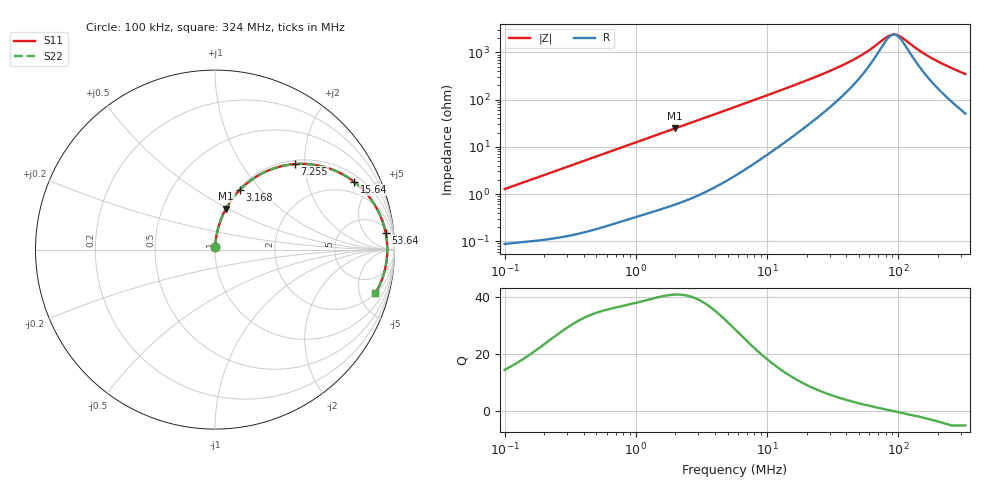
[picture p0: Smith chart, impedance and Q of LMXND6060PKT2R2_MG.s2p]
! LMXND6060PKT2R2_MG  S-PARAMETER MODEL  ( General Type )
! Model Generated by TAIYO YUDEN Corporation (https://www.yuden.co.jp/en/)
! Version 1.0
! TAIYO YUDEN Control No. 191025NI43SB-FBB
! Copyright(c) 2019 TAIYO YUDEN CO.,LTD. All Rights Reserved.
! Product Description (link to TY-COMPAS)
! https://ds.yuden.co.jp/TYCOMPAS/or/detail?pn=LMXND6060PKT2R2NMG&u=M
! Products Name : Inductors
! Characteristics :
!  Inductance : 2.2 uH , SRF(min) : 61 MHz , DC Resistance(max) : 0.066 Ohm
!  Rated Current : Saturation :3000 mA , Temp Rise : 2300 mA (40 degC)
!  Case Size : 6.0 x 6.0 / 0.236 x 0.236 [mm/inch] , Thickness : 1.4 / 0.055 [mm/inch]
!  (Conditions: Temperature = 25 degC , DC Bias Current/Voltage = 0A / 0V)
! External Node Assignments :
!  1  o---GGG---o  2
! GND o---------o GND
! Frequency Range : 0.1MHz  -  324.04089MHz  [ 402 STEP ]
# MHz S RI R 50
! Freq[MHz].  S11 Real  S11 Imag  S21 Real  S21 Imag  S12 Real  S12 Imag  S22 Real  S22 Imag
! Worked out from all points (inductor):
!   401 points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, 100 kHz to 324 MHz, reference 50 ohm
!   read as one part in series: L = 2.02 uH near 104.1 kHz
!   highest Q = 40.9 at 1.99 MHz (marker M1), where L = 1.95 uH
!   self-resonance near 92.57 MHz
!   S11 on the Smith chart (normalised r, x): 100 kHz: 1.00, +0.03; 3.168 MHz: 1.02, +0.78; 7.255 MHz: 1.07, +1.78; 15.64 MHz: 1.33, +3.91; 53.64 MHz: 8, +17; 324 MHz: 2.01, -6.89
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0.1  0.00104 0.0127  0.999 -0.0127  0.999 -0.0127  0.00104 0.0127
0.38728  0.00383 0.0482  0.9962 -0.0482  0.9962 -0.0482  0.00383 0.0482
0.80164  0.0124 0.098  0.9876 -0.098  0.9876 -0.098  0.0124 0.098
1.499861  0.0371 0.177  0.9629 -0.177  0.9629 -0.177  0.0371 0.177
1.990316  0.0613 0.228  0.9387 -0.228  0.9387 -0.228  0.0613 0.228
3.167973  0.1373 0.3315  0.8627 -0.3315  0.8627 -0.3315  0.1373 0.3315
4.2039  0.2164 0.3976  0.7836 -0.3976  0.7836 -0.3976  0.2164 0.3976
5.692459  0.3332 0.4543  0.6668 -0.4543  0.6668 -0.4543  0.3332 0.4543
7.254674  0.4451 0.4766  0.5549 -0.4766  0.5549 -0.4766  0.4451 0.4766
10.22865  0.609 0.4608  0.391 -0.4608  0.391 -0.4608  0.609 0.4608
15.63597  0.7748 0.3778  0.2252 -0.3778  0.2252 -0.3778  0.7748 0.3778
22.04577  0.8622 0.2897  0.1378 -0.2897  0.1378 -0.2897  0.8622 0.2897
36.53742  0.9292 0.1686  0.0708 -0.1686  0.0708 -0.1686  0.9292 0.1686
53.64032  0.9509 0.0925  0.0491 -0.0925  0.0491 -0.0925  0.9509 0.0925
85.37896  0.9598 0.0132  0.0402 -0.0132  0.0402 -0.0132  0.9598 0.0132
92.56714  0.96 9.66e-06  0.04 -9.66e-06  0.04 -9.66e-06  0.96 9.66e-06
100.3605  0.9598 -0.0132  0.0402 0.0132  0.0402 0.0132  0.9598 -0.0132
108.81  0.9593 -0.0264  0.0407 0.0264  0.0407 0.0264  0.9593 -0.0264
144.3909  0.9542 -0.0744  0.0458 0.0744  0.0458 0.0744  0.9542 -0.0744
176.7278  0.9469 -0.1113  0.0531 0.1113  0.0531 0.1113  0.9469 -0.1113
239.3053  0.9277 -0.1731  0.0723 0.1731  0.0723 0.1731  0.9277 -0.1731
324.0409  0.8935 -0.2438  0.1065 0.2438  0.1065 0.2438  0.8935 -0.2438
